DATA_BLOCK DB 1
TITLE =
VERSION : 0.1


  STRUCT
   DB_VAR : INT:= 50 ;	//Temporary placeholder variable
   DB_VAR2 : REAL  := 6.000000e+001;	//dk
  END_STRUCT ;
BEGIN
   DB_VAR := 0;
   DB_VAR2 := 5.000000e+001;
END_DATA_BLOCK

